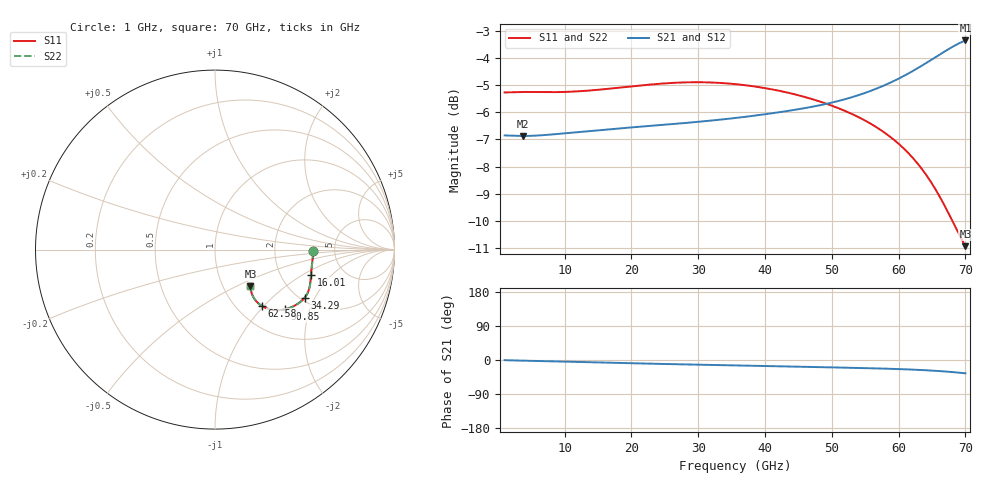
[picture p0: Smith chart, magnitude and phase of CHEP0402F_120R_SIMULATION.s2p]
! Touchstone file exported from HFSS 2026.1.0
!  File:  S:/COMPOSANTS_3D_CRYPTES/CHEP0402F/2026R1/PCB_&_COMP/PCB_V1.1.003_CHEP0402F_V1.aedt
!  $RV = 120ohm
# GHz S MA R 50.000000
! Terminal data exported
! Port[1] = LINE_T1
! Port[2] = LINE_T2
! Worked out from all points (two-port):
!   401 points, 1 GHz to 70 GHz, reference 50 ohm
!   highest |S21| = -3.34 dB at 70 GHz (marker M1); lowest = -6.9 dB at 3.76 GHz (marker M2)
!   |S21| within 3 dB of the highest: 30.25 GHz to end of sweep
!   lowest |S11| = -10.9 dB at 70 GHz (marker M3), VSWR 1.79, Z = 67.1 - j29.7 ohm
!   |S11| at or under -10 dB: 68.03 GHz to end of sweep
!   |S22| runs from -11.0 to -4.9 dB; largest |S21 - S12| = 1e-14
!   S11 on the Smith chart (normalised r, x): 1 GHz: 3.40, -0.09; 16.01 GHz: 2.94, -1.20; 34.29 GHz: 2.11, -1.66; 50.85 GHz: 1.52, -1.37; 62.58 GHz: 1.29, -0.97; 70 GHz: 1.34, -0.59
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1  0.5456 -1.0  0.4544 -0.5  0.4544 -0.5  0.5456 -1.0
3.76  0.5466 -3.7  0.4534 -1.7  0.4534 -1.7  0.5467 -3.7
7.3825  0.5463 -7.2  0.4556 -3.1  0.4556 -3.1  0.5465 -7.3
12.5575  0.5488 -11.9  0.4617 -5.3  0.4617 -5.3  0.5492 -11.9
16.0075  0.5533 -14.8  0.4658 -6.8  0.4658 -6.8  0.5538 -14.8
24.115  0.566 -21.2  0.4746 -10.2  0.4746 -10.2  0.5664 -21.2
29.29  0.5698 -24.9  0.4806 -12.1  0.4806 -12.1  0.57 -24.8
34.2925  0.567 -28.2  0.4875 -13.9  0.4875 -13.9  0.567 -28.2
35.5  0.5653 -29.0  0.4893 -14.3  0.4893 -14.3  0.5652 -29.0
41.1925  0.5523 -32.9  0.4997 -16.3  0.4997 -16.3  0.5521 -33.0
44.125  0.5425 -35.2  0.506 -17.3  0.506 -17.3  0.5422 -35.2
47.0575  0.5303 -37.5  0.5133 -18.4  0.5133 -18.4  0.5302 -37.6
50.8525  0.511 -40.7  0.5256 -19.8  0.5256 -19.8  0.511 -40.7
54.9925  0.484 -44.3  0.5446 -21.4  0.5446 -21.4  0.4841 -44.3
58.615  0.453 -47.4  0.5677 -23.1  0.5677 -23.1  0.4531 -47.4
60.685  0.4309 -49.0  0.5844 -24.4  0.5844 -24.4  0.431 -49.1
62.5825  0.4069 -50.3  0.6022 -25.7  0.6022 -25.7  0.4069 -50.4
64.3075  0.3814 -51.2  0.6203 -27.2  0.6203 -27.2  0.3814 -51.2
66.0325  0.3524 -51.3  0.6397 -29.1  0.6397 -29.1  0.3523 -51.3
68.1025  0.315 -49.8  0.6628 -31.9  0.6628 -31.9  0.3148 -49.8
69.655  0.2889 -46.7  0.6778 -34.5  0.6778 -34.5  0.2886 -46.7
70  0.2837 -45.8  0.6806 -35.1  0.6806 -35.1  0.2834 -45.8
